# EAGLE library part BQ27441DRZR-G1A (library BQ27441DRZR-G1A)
System-Side Impedance Track Battery Fuel (Gas) Gauge Source: Datasheet
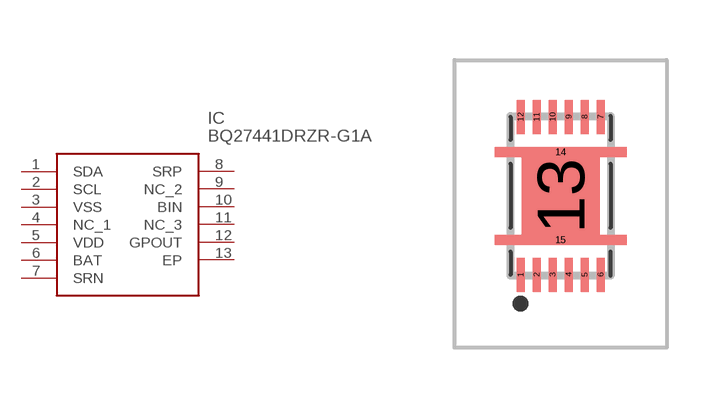
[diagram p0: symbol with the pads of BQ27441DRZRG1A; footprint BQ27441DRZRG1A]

Designator prefix IC

## BQ27441DRZR-G1A (Arrow_Part_Number: BQ27441DRZR-G1A; Arrow_Price-Stock: https://www.arrow.com/en/products/bq27441drzr-g1a/texas-instruments; Description: System-Side Impedance Track Battery Fuel (Gas) Gauge; Height: mm; Manufacturer_Name: Texas Instruments; Manufacturer_Part_Number: BQ27441DRZR-G1A)  [BQ27441DRZRG1A]
1  SDA
2  SCL
3  VSS
4  NC_1
5  VDD
6  BAT
7  SRN
8  SRP
9  NC_2
10  BIN
11  NC_3
12  GPOUT
13  EP

## Footprint BQ27441DRZRG1A (pad centres in mm)
DRZ (S-PDSO-N12)
smd 0.2 x 0.85: 1 -1,-1.975; 2 -0.6,-1.975; 3 -0.2,-1.975; 4 0.2,-1.975; 5 0.6,-1.975; 6 1,-1.975; 7 1,1.975; 8 0.6,1.975; 9 0.2,1.975; 10 -0.2,1.975; 11 -0.6,1.975; 12 -1,1.975
smd 1.95 x 1.95: 13 0,0
smd 3.3 x 0.25: 14 0,1.1; 15 0,-1.1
